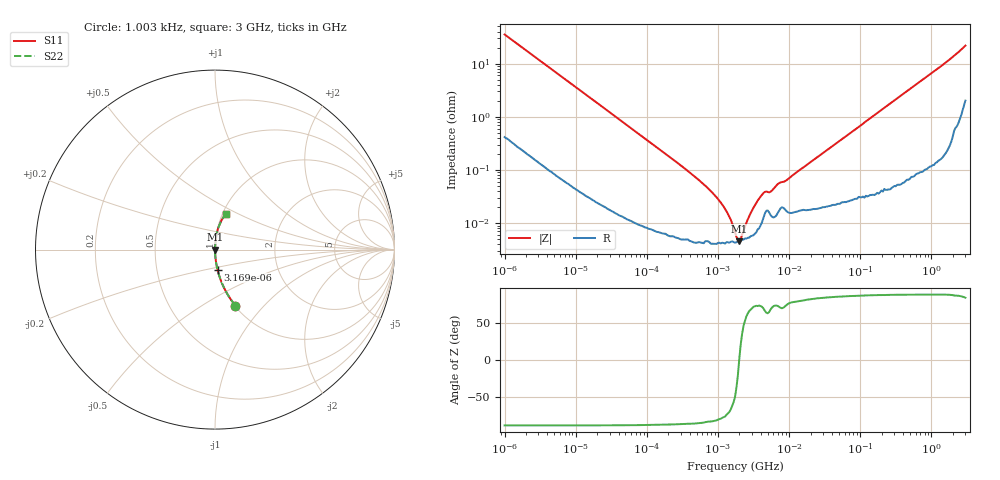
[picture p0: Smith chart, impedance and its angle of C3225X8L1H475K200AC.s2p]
! S-Parameter Data Generated by TDK Corporation
! Copyright(C) 2022 TDK Corporation.
! All Rights Reserved.
! TDK P/N: C3225X8L1H475K200AC (Multilayer Ceramic Chip Capacitor)
! Property: C=4.7uF
! Size(LxWxT): 3.2x2.5x2mm
! Model Type: s2p (Touchstone File Format Version 1.0)
! Frequency: DC=Yes Start=0.00100273MHz Stop=3000MHz 326points Log-sweep
! Model Generated on Apr. 15, 2022
! Port Assignments:
!  1 ---| |--- 2
! Applicable Conditions:
!  Temperature = 25 degC
!  DC Bias Voltage = 0 V
!  Small Signal Operation
! Terms and conditions regarding TDK Simulation Models
! (1)This simulation model is being provided solely for informational purposes. Please refer to the specifications of the products in terms of detailed characteristics of such products.
! (2)In no event shall TDK Corporation of any of its subsidiaries be liable for any loss or damage arising, directly or indirectly,
!  From any information contained in this simulation model, including, but not limited to loss or damages arising from any inaccuracies, omissions or errors in connection with such information.
! (3)Any and all copyrights on this simulation model are owned by TDK Corporation.
!  Duplication or redistribution of this simulation model without prior written permission from TDK Corporation is prohibited.
! (4)This simulation model is subject to any modification or change without any prior notice.
! (5)Neither TDK Corporation nor any of its subsidiaries shall make any warranty, express or implied,
!  Including but not limited to the correctness, implied warranties of merchantability and fitness for a particular purpose with respect to this simulation models.
! (6)The use of this simulation model shall be deemed to have consented to the terms and conditions hereof.
# Hz S MA R 50
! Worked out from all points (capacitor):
!   325 points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, 1.003 kHz to 3 GHz, reference 50 ohm
!   read as one part in series: C = 4.47 uF near 1.05 kHz
!   lowest |Z| = 4.55 mohm at 1.991 MHz (marker M1)
!   series resonance near 1.988 MHz, so ESL is about 1.4 nH
!   S11 on the Smith chart (normalised r, x): 1.003 kHz: 1.01, -0.71; 3.169 kHz: 1.00, -0.23; 3 GHz: 1.04, +0.43
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1002.73  0.3323 -69.9  0.9393 19.4  0.9393 19.4  0.3323 -69.9
1663.58  0.2092 -77.3  0.9754 12.1  0.9754 12.1  0.2092 -77.3
3168.61  0.1125 -82.9  0.9924 6.5  0.9924 6.5  0.1125 -82.9
12036.7  0.03017 -87.6  0.9992 1.7  0.9992 1.7  0.03017 -87.6
151292  0.002443 -88.3  0.9999 0.1  0.9999 0.1  0.002443 -88.3
690880  0.0004803 -84.5  1 0.0  1 0.0  0.0004803 -84.5
1094650  0.000244 -80.2  1 0.0  1 0.0  0.000244 -80.2
1315910  0.0001672 -74.9  1 0.0  1 0.0  0.0001672 -74.9
1581890  9.911e-05 -62.8  1 0.0  1 0.0  9.911e-05 -62.8
1816100  5.53e-05 -38.0  1 0.0  1 0.0  5.53e-05 -38.0
1991200  4.547e-05 0.9  1 -0.0  1 -0.0  4.547e-05 0.9
2506410  0.0001004 59.3  0.9999 -0.0  0.9999 -0.0  0.0001004 59.3
3154920  0.0001951 72.3  0.9999 -0.0  0.9999 -0.0  0.0001951 72.3
4354130  0.0003692 70.1  0.9999 -0.0  0.9999 -0.0  0.0003692 70.1
4773930  0.0003934 64.3  0.9998 -0.0  0.9998 -0.0  0.0003934 64.3
5480730  0.0003886 68.6  0.9999 -0.0  0.9999 -0.0  0.0003886 68.6
6898840  0.0005415 73.4  0.9998 -0.0  0.9998 -0.0  0.0005415 73.4
9092860  0.0006345 74.3  0.9998 -0.0  0.9998 -0.0  0.0006345 74.3
2.18003e7  0.00153 83.0  0.9998 -0.1  0.9998 -0.1  0.00153 83.0
2.61689e8  0.01771 87.6  0.9994 -1.0  0.9994 -1.0  0.01771 87.6
1.19501e9  0.07823 84.5  0.9955 -4.5  0.9955 -4.5  0.07823 84.5
3e9  0.2089 72.7  0.9588 -12.0  0.9588 -12.0  0.2089 72.7
